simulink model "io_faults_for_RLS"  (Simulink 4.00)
settings: Solver=ode45  StartTime=0.0  StopTime=1020  RelTol=1e-3
libraries: simulink3 x2

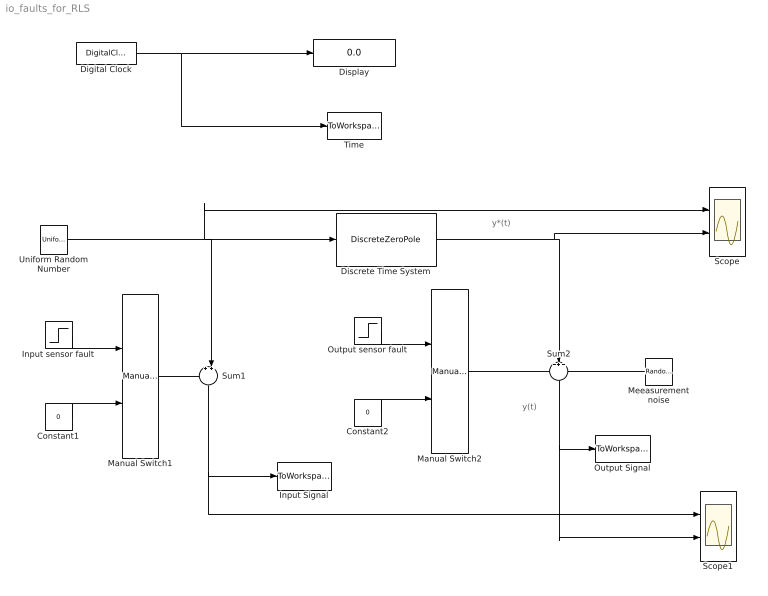
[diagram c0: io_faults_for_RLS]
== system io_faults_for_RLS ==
  note: y*(t)
  note: y(t)
  Constant1 : Constant  Value=0
  Constant2 : Constant  Value=0
  Digital Clock : DigitalClock  SampleTime=1
  Discrete Time System : DiscreteZeroPole  Zeros=[]  Poles=[0.6 0.7 0.8]  Gain=0.0240  SampleTime=1
  Display : Display
  Input Signal : ToWorkspace  VariableName=U  SampleTime=1  SaveFormat=Array
  Input sensor fault : Step  Time=500  Before=0  After=-1  SampleTime=1
  Manual Switch1 : simulink3/Nonlinear/Manual Switch  sw=0  action=0
  Manual Switch2 : simulink3/Nonlinear/Manual Switch  sw=0  action=0
  Meeasurement noise : RandomNumber  Orientation=left  Mean=0  Variance=(0.01)^2  Seed=3  SampleTime=1
  Output Signal : ToWorkspace  VariableName=Y  SampleTime=1  SaveFormat=Array
  Output sensor fault : Step  Time=500  Before=0  After=1  SampleTime=0
  Scope : Scope  NumInputPorts=2
  Scope1 : Scope  NumInputPorts=2
  Sum1 : Sum  Orientation=down  Inputs=++|  SaturateOnIntegerOverflow=on
  Sum2 : Sum  Orientation=down  Inputs=+++  SaturateOnIntegerOverflow=on
  Time : ToWorkspace  VariableName=t  SampleTime=1  SaveFormat=Array
  Uniform Random Number : UniformRandomNumber  Minimum=-1  Maximum=1  Seed=0  SampleTime=1
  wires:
  Digital Clock/1 -> Display/1, Time/1
  Uniform Random Number/1 -> Sum1/2, Scope/1, Discrete Time System/1
  Discrete Time System/1 -> Scope/2, Sum2/2
  Constant1/1 -> Manual Switch1/2
  Sum1/1 -> Input Signal/1, Scope1/1
  Manual Switch1/1 -> Sum1/1
  Input sensor fault/1 -> Manual Switch1/1
  Constant2/1 -> Manual Switch2/2
  Manual Switch2/1 -> Sum2/1
  Output sensor fault/1 -> Manual Switch2/1
  Sum2/1 -> Output Signal/1, Scope1/2
  Meeasurement noise/1 -> Sum2/3
